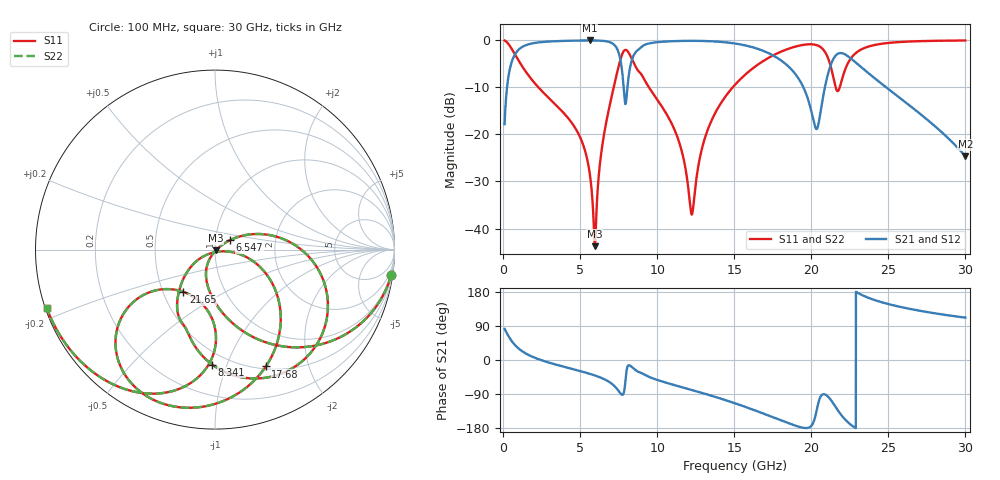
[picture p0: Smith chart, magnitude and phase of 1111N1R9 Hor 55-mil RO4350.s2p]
# GHz S MA R 50
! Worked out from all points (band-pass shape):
!   3201 points, 100 MHz to 30 GHz, reference 50 ohm
!   highest |S21| = -0.05 dB at 5.631 GHz (marker M1); lowest = -24.7 dB at 30 GHz (marker M2)
!   |S21| within 3 dB of the highest: 766 MHz to 7.537 GHz (6.771 GHz wide, 163 % of centre); 8.502 GHz to 17.41 GHz (8.911 GHz wide, 68.8 % of centre)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
!   lowest |S11| = -43.8 dB at 5.959 GHz (marker M3), VSWR 1.01, Z = 50.5 - j0.429 ohm
!   |S11| at or under -10 dB: 2.29 GHz to 7.18 GHz (4.89 GHz wide, 103 % of centre); 9.464 GHz to 14.91 GHz (5.442 GHz wide, 44.7 % of centre); 21.58 GHz to 21.85 GHz (269.6 MHz wide, 1.24 % of centre)
!   |S22| runs from -43.8 to -0.1 dB; largest |S21 - S12| = 0
!   S11 on the Smith chart (normalised r, x): 100 MHz: 1, -14; 6.547 GHz: 1.18, +0.12; 8.341 GHz: 0.41, -0.89; 17.68 GHz: 0.53, -1.39; 21.65 GHz: 0.63, -0.33; 30 GHz: 0.00, -0.17
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0.1  0.9917 -8.1  0.1284 81.9  0.1284 81.9  0.9917 -8.1
0.6045625  0.7873 -42.3  0.6159 47.7  0.6159 47.7  0.7873 -42.3
1.679094  0.4169 -77.0  0.9075 12.8  0.9075 12.8  0.4169 -77.0
5.089563  0.0861 -117.8  0.9922 -30.2  0.9922 -30.2  0.0861 -117.8
5.6315  0.03766 -119.0  0.9937 -36.6  0.9937 -36.6  0.03766 -119.0
5.958531  0.006491 -40.9  0.9928 -40.8  0.9928 -40.8  0.006491 -40.9
6.547187  0.09891 32.1  0.9813 -50.3  0.9813 -50.3  0.09891 32.1
7.715156  0.6995 -25.9  0.4827 -91.8  0.4827 -91.8  0.6995 -25.9
7.967437  0.7893 -56.6  0.2149 -42.7  0.2149 -42.7  0.7893 -56.6
8.341188  0.6409 -91.3  0.6039 -18.1  0.6039 -18.1  0.6409 -91.3
10.06978  0.2254 -138.7  0.9546 -53.5  0.9546 -53.5  0.2254 -138.7
11.44331  0.0809 -149.7  0.9812 -70.0  0.9812 -70.0  0.0809 -149.7
12.24687  0.01405 -79.0  0.9847 -79.1  0.9847 -79.1  0.01405 -79.0
13.21862  0.1049 -8.6  0.9786 -90.6  0.9786 -90.6  0.1049 -8.6
15.05  0.3362 -27.3  0.9223 -114.2  0.9223 -114.2  0.3362 -27.3
17.67559  0.71 -66.5  0.6662 -153.5  0.6662 -153.5  0.71 -66.5
20.03956  0.905 -111.7  0.1658 -171.9  0.1658 -171.9  0.905 -111.7
20.93656  0.7287 -139.2  0.3483 -91.8  0.3483 -91.8  0.7287 -139.2
21.64669  0.2941 -126.8  0.7038 -128.0  0.7038 -128.0  0.2941 -126.8
23.02956  0.7605 -100.7  0.5535 176.8  0.5535 176.8  0.7605 -100.7
25.01978  0.9356 -125.5  0.3013 147.4  0.3013 147.4  0.9356 -125.5
30  0.9926 -160.9  0.05851 111.8  0.05851 111.8  0.9926 -160.9
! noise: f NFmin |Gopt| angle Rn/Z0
0.1  0.001852  0.911  2.983  0.004572
3.417  0.01157  0.5437  26.18  0.004296
6.743  0.04655  0.7527  45.55  0.03241
10.06  0.05771  0.7184  67.17  0.02848
13.39  0.05801  0.6521  84.86  0.01792
16.7  0.09355  0.7283  101.2  0.02864
20.03  0.8972  0.9618  119.7  1.349
23.35  0.2459  0.8504  134.3  0.05473
26.67  0.3132  0.8801  147.5  0.04643
30  0.7348  0.9496  162.5  0.07806
